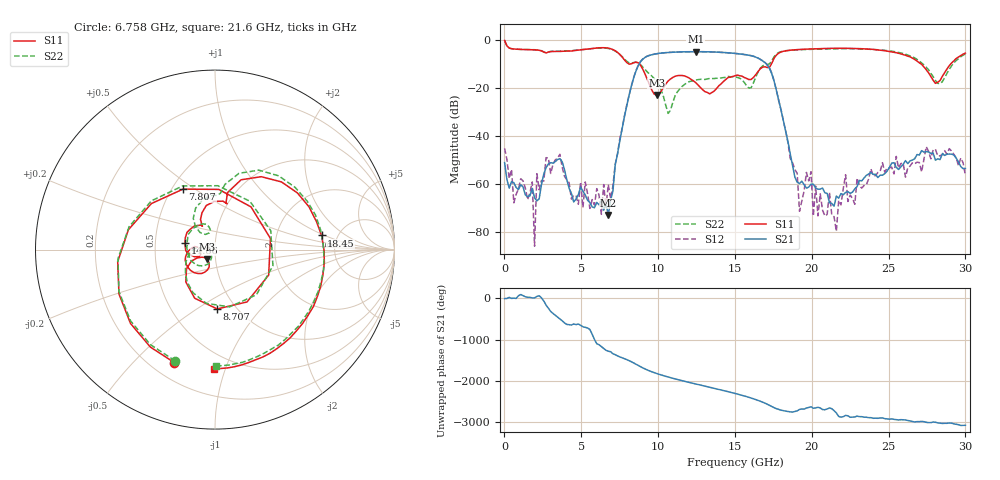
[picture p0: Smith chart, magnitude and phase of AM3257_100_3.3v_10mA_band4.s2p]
!Keysight Technologies,N5245B,MY58422270,A.16.20.02
!Date: Wednesday, June 18, 2025 22:47:25
!Correction: S11(C  2-Port  )
!S21(C  2-Port  )
!S12(C  2-Port  )
!S22(C  2-Port  )
!S2P File: Measurements: S11, S21, S12, S22:
# Hz S  dB  R 50
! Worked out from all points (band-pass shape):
!   201 points, 10 MHz to 30 GHz, reference 50 ohm
!   highest |S21| = -4.96 dB at 12.46 GHz (marker M1); lowest = -73.1 dB at 6.758 GHz (marker M2)
!   |S21| within 3 dB of the highest: 9.028 GHz to 16.59 GHz (7.563 GHz wide, 59 % of centre)
!   lowest |S11| = -23.0 dB at 9.907 GHz (marker M3), VSWR 1.15, Z = 45.4 - j5 ohm
!   |S11| at or under -10 dB: 8.076 GHz to 8.268 GHz (192 MHz wide, 2.35 % of centre); 8.764 GHz to 17.38 GHz (8.619 GHz wide, 65.9 % of centre); 27.1 GHz to 29.06 GHz (1.96 GHz wide, 6.98 % of centre)
!   |S22| runs from -30.7 to -0.3 dB; largest |S21 - S12| = 0.0097
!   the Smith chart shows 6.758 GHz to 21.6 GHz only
!   S11 on the Smith chart (normalised r, x): 6.758 GHz: 0.29, -0.66; 7.807 GHz: 0.57, +0.45; 8.707 GHz: 0.82, -0.61; 14.86 GHz: 0.71, +0.06; 18.45 GHz: 3.75, +0.92; 21.6 GHz: 0.39, -0.92
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1e7  -0.29 -9.6  -51.20 -12.7  -45.22 -48.8  -0.29 -9.9
6.098e8  -3.85 -173.4  -59.60 -0.4  -67.97 -44.2  -3.85 -173.7
1.8094e9  -4.14 134.1  -61.94 4.3  -59.25 -1.4  -4.11 134.0
1.95935e9  -4.19 128.4  -65.87 5.6  -86.02 -79.9  -4.15 128.3
2.1093e9  -4.26 122.4  -67.16 40.1  -55.82 -31.7  -4.22 122.4
3.6088e9  -4.86 72.0  -49.55 -142.6  -47.73 -141.7  -4.77 72.7
5.1083e9  -4.12 3.6  -63.16 27.4  -69.90 -80.5  -4.10 5.1
6.75775e9  -3.49 -109.7  -73.05 157.2  -60.31 -89.0  -3.63 -109.7
7.8074e9  -8.38 117.9  -32.14 -22.2  -31.77 -22.3  -8.01 116.9
8.7071e9  -9.61 -87.9  -10.81 173.6  -10.60 173.5  -9.64 -75.7
9.9067e9  -23.00 -129.3  -5.81 -20.8  -5.77 -20.9  -17.31 -174.6
1.005665e10  -22.57 -119.8  -5.66 -39.0  -5.63 -39.2  -18.85 176.9
1.245585e10  -17.91 175.2  -4.96 85.5  -4.97 85.4  -16.79 -152.6
1.485505e10  -15.29 167.0  -5.59 -127.5  -5.58 -127.4  -15.40 138.0
1.5005e10  -14.99 158.4  -5.68 -141.8  -5.66 -141.7  -15.53 130.4
1.725425e10  -11.42 76.8  -12.00 -69.9  -11.69 -69.2  -10.02 84.5
1.845385e10  -4.45 7.5  -42.45 141.8  -43.05 144.3  -4.46 10.8
2.01033e10  -3.77 -53.9  -60.20 -139.6  -73.48 -122.4  -3.95 -52.0
2.16028e10  -3.55 -90.3  -65.13 107.4  -79.81 -46.0  -3.75 -89.6
2.22026e10  -3.55 -102.4  -63.60 47.1  -56.24 33.1  -3.72 -102.1
2.505165e10  -4.87 -158.0  -53.24 -44.2  -53.39 -20.6  -4.64 -157.4
3e10  -5.56 -86.0  -53.65 169.0  -56.59 -159.6  -5.93 -87.6
